[IBIS VER]   4.1
[File Name]   f28p55xpbk.ibs
[File Rev]   2.0
[Date]   August 28, 2024
[Source]   File originated at Texas Instruments
[Copyright]   (c) 2012, Texas Instruments Inc.
[Component]   f28p55xpbk
[Manufacturer]  Texas Instruments
[Package]
| Variable   Typ   Min   Max
R_pkg  3.39E-01  1.39E-01  3.88E-01
L_pkg  6.91E-09  4.87E-09  8.02E-09
C_pkg  9.61E-15  7.42E-15  1.07E-14
[Pin]   signal_name   model_name   R_pin   L_pin   C_pin
   1   GPIO29   BCF3385DSHYPBFZ_LC  3.76E-01  7.81E-09  1.01E-14
   2   A16,B16,C16,GPIO28   BCF3385DSHYPBFZ_LC  3.69E-01  7.66E-09  9.95E-15
   3   XRSn   BQ0491FS_USF  3.59E-01  7.49E-09  9.73E-15
   4   GPIO46   BCF3385DSHYPBFZ_LC  3.51E-01  7.33E-09  9.53E-15
   5   VDDIO   NC  3.49E-01  7.23E-09  9.37E-15
   6   VDD   NC  1.87E-01  5.49E-09  8.01E-15
   7   VSS   NC  1.86E-01  5.40E-09  7.86E-15
   8   GPIO47   BCF3385DSHYPBFZ_LC_USF  3.37E-01  6.88E-09  8.87E-15
   9   GPIO66   BCF3385DSHYPBFZ_LC_USF  3.33E-01  6.76E-09  1.03E-14
   10   GPIO67   BCF3385DSHYPBFZ_LC_USF  3.30E-01  6.66E-09  1.01E-14
   11   GPIO48   BCF3385DSHYPBFZ_LC_USF  3.28E-01  6.57E-09  9.90E-15
   12   GPIO49   BCF3385DSHYPBFZ_LC_USF  3.27E-01  6.48E-09  9.72E-15
   13   GPIO50   BCF3385DSHYPBFZ_LC_USF  3.27E-01  6.41E-09  9.55E-15
   14   GPIO51   BCF3385DSHYPBFZ_LC_USF  3.29E-01  6.35E-09  9.38E-15
   15   GPIO52   BCF3385DSHYPBFZ_LC_USF  3.31E-01  6.29E-09  9.22E-15
   16   GPIO53   BCF3385DSHYPBFZ_LC_USF  3.34E-01  6.25E-09  9.07E-15
   17   GPIO54   BCF3385DSHYPBFZ_LC_USF  3.36E-01  6.27E-09  9.09E-15
   18   A6,D14,E14,GPIO228   BCF3385DSHYPBFZ_LC_USF  3.36E-01  6.35E-09  9.26E-15
   19   B2,C6,E12,GPIO226   BCF3385DSHYPBFZ_LC_USF  3.37E-01  6.44E-09  9.45E-15
   20   A3,B3,C5,GPIO242,PGA2_INP   BCF3385DSHYPBFZ_LC_USF  3.58E-01  6.72E-09  9.78E-15
   21   A2,B6,C9,GPIO224,PGA1_INP   BCF3385DSHYPBFZ_LC  3.37E-01  6.58E-09  9.79E-15
   22   A15,B9,C7,PGA1_INM   ICF33SHYPB_LC  3.31E-01  6.59E-09  9.92E-15
   23   C25,D5,E5   ICF33SHYPB_LC  3.29E-01  6.65E-09  1.01E-14
   24   A26,D6,E6   ICF33SHYPB_LC  3.32E-01  6.76E-09  1.03E-14
   25   B26,D7,E7   ICF33SHYPB_LC  3.36E-01  6.87E-09  8.86E-15
   26   A14,B14,C4,PGA1_OUT   ICF33SHYPB_LC  3.40E-01  6.99E-09  9.03E-15
   27   A11,B10,C0,PGA2_OUT   ICF33SHYPB_LC  3.46E-01  7.13E-09  9.22E-15
   28   A5,B12,C2,PGA2_INM   ICF33SHYPB_LC  3.62E-01  7.36E-09  9.47E-15
   29   A1,B7,D11,DACB_OUT   ICF33SHYPB_LC  3.58E-01  7.39E-09  9.58E-15
   30   A0,B15,C15,DACA_OUT   ICF33SHYPB_LC  3.67E-01  7.56E-09  9.79E-15
   31   D20,E20,VREFHI   ICF33SHYPB_LC  3.73E-01  7.70E-09  9.97E-15
   32   D20,E20,VREFHI   ICF33SHYPB_LC  2.06E-01  6.06E-09  8.85E-15
   33   A13,B13,C13,D13,E13,VREFLO   ICF33SHYPB_LC  3.84E-01  8.02E-09  1.04E-14
   34   A13,B13,C13,D13,E13,VREFLO   ICF33SHYPB_LC  2.04E-01  6.08E-09  8.91E-15
   35   A12,C1,E11,PGA3_INP   ICF33SHYPB_LC  3.74E-01  7.75E-09  1.01E-14
   36   B11,D16,E16,PGA3_INM   ICF33SHYPB_LC  3.70E-01  7.63E-09  9.88E-15
   37   A7,B30,C3,D12,E30   ICF33SHYPB_LC  3.66E-01  7.52E-09  9.71E-15
   38   B5,D15,E15,PGA3_OUT   ICF33SHYPB_LC  3.69E-01  7.47E-09  9.59E-15
   39   A8,B0,C11   ICF33SHYPB_LC  3.59E-01  7.29E-09  9.37E-15
   40   VSSA   NC  1.40E-01  4.96E-09  7.57E-15
   41   VDDA   NC  1.39E-01  4.87E-09  7.42E-15
   42   A4,B8,C14   ICF33SHYPB_LC  3.65E-01  7.13E-09  1.06E-14
   43   C26,D8,E8,GPIO211   BCF3385DSHYPBFZ_LC  3.75E-01  7.15E-09  1.05E-14
   44   A27,D9,E9,GPIO212   BCF3385DSHYPBFZ_LC  3.71E-01  7.03E-09  1.03E-14
   45   B27,D10,E10,GPIO213   BCF3385DSHYPBFZ_LC  3.67E-01  6.91E-09  1.01E-14
   46   C27,D18,E18,GPIO214   BCF3385DSHYPBFZ_LC  3.65E-01  6.81E-09  9.87E-15
   47   A28,D19,E19,GPIO215   BCF3385DSHYPBFZ_LC  3.63E-01  6.72E-09  9.67E-15
   48   A9,GPIO227   BCF3385DSHYPBFZ_LC  3.62E-01  6.63E-09  9.49E-15
   49   B4,C8,GPIO236   BCF3385DSHYPBFZ_LC  3.60E-01  6.60E-09  9.47E-15
   50   A10,B1,C10,GPIO230   BCF3385DSHYPBFZ_LC  3.56E-01  6.65E-09  9.62E-15
   51   GPIO55   BCF3385DSHYPBFZ_LC  3.54E-01  6.70E-09  9.78E-15
   52   GPIO60   BCF3385DSHYPBFZ_LC  3.51E-01  6.75E-09  9.94E-15
   53   VSS   NC  1.90E-01  5.17E-09  8.90E-15
   54   VDD   NC  1.89E-01  5.24E-09  9.07E-15
   55   VDDIO   NC  3.51E-01  6.98E-09  1.05E-14
   56   GPIO64   BCF3385DSHYPBFZ_LC  3.46E-01  7.00E-09  8.99E-15
   57   GPIO65   BCF3385DSHYPBFZ_LC  3.47E-01  7.09E-09  9.14E-15
   58   GPIO62   BCF3385DSHYPBFZ_LC  3.49E-01  7.19E-09  9.30E-15
   59   GPIO63   BCF3385DSHYPBFZ_LC  3.52E-01  7.29E-09  9.46E-15
   60   A17,B17,C17,GPIO20   BCF3385DSHYPBFZ_LC  3.56E-01  7.42E-09  9.64E-15
   61   A18,B18,C18,GPIO21   BCF3385DSHYPBFZ_LC  3.61E-01  7.55E-09  9.82E-15
   62   A19,B19,C19,GPIO13   BCF3385DSHYPBFZ_LC  3.68E-01  7.69E-09  1.00E-14
   63   A20,B20,C20,GPIO12   BCF3385DSHYPBFZ_LC  3.76E-01  7.85E-09  1.02E-14
   64   A24,D0,E0,GPIO11   BCF3385DSHYPBFZ_LC  3.81E-01  7.98E-09  1.04E-14
   65   B24,D1,E1,GPIO33   BCF3385DSHYPBFZ_LC  3.80E-01  7.85E-09  1.02E-14
   66   C24,D2,E2,GPIO16   BCF3385DSHYPBFZ_LC  3.69E-01  7.66E-09  9.94E-15
   67   A25,D3,E3,GPIO17   BCF3385DSHYPBFZ_LC  3.60E-01  7.49E-09  9.73E-15
   68   B25,D4,E4,GPIO24   BCF3385DSHYPBFZ_LC  3.51E-01  7.33E-09  9.54E-15
   69   GPIO25   BCF3385DSHYPBFZ_LC  3.48E-01  7.22E-09  9.37E-15
   70   GPIO26   BCF3385DSHYPBFZ_LC  3.42E-01  7.08E-09  9.18E-15
   71   GPIO27   BCF3385DSHYPBFZ_LC  3.40E-01  6.98E-09  9.03E-15
   72   GPIO68   BCF3385DSHYPBFZ_LC  3.36E-01  6.87E-09  8.86E-15
   73   GPIO69   BCF3385DSHYPBFZ_LC  3.33E-01  6.76E-09  1.03E-14
   74   GPIO70   BCF3385DSHYPBFZ_LC  3.31E-01  6.67E-09  1.01E-14
   75   TCK   BCF3355DSHYPBFZ_TMS_USF  3.30E-01  6.59E-09  9.92E-15
   76   GPIO37/TDO   BCPF335585DSHYPBFZ  3.30E-01  6.52E-09  9.74E-15
   77   TMS   BCF3355DSHYPBFZ_TMS  3.32E-01  6.45E-09  9.58E-15
   78   GPIO35/TDI   BCF3385DSHYPBFZ_LC  3.34E-01  6.40E-09  9.42E-15
   79   GPIO32   BQ33100HYPBFZ_PMB_5FS_LC  3.36E-01  6.35E-09  9.27E-15
   80   GPIO56   BCF3385DSHYPBFZ_LC  3.39E-01  6.30E-09  9.11E-15
   81   GPIO57   BCF3385DSHYPBFZ_LC  3.41E-01  6.32E-09  9.12E-15
   82   GPIO58   BCF3385DSHYPBFZ_LC  3.41E-01  6.40E-09  9.30E-15
   83   GPIO71   BCF3385DSHYPBFZ_LC  3.42E-01  6.49E-09  9.49E-15
   84   GPIO72   BCF3385DSHYPBFZ_LC  3.45E-01  6.59E-09  9.68E-15
   85   GPIO73   BCF3385DSHYPBFZ_LC  3.48E-01  6.69E-09  9.87E-15
   86   GPIO74   BCF3385DSHYPBFZ_LC  3.52E-01  6.81E-09  1.01E-14
   87   GPIO18,X2   BCF3385DSHYPBFZ_LC  3.66E-01  7.03E-09  1.04E-14
   88   GPIO19,X1   BCPF335585DSHYPBFZ  3.51E-01  6.95E-09  1.04E-14
   89   VDDIO   NC  3.59E-01  7.11E-09  9.04E-15
   90   VDD   NC  1.89E-01  5.43E-09  7.88E-15
   91   GPIO43   BCF3385DSHYPBFZ_LC  3.54E-01  7.21E-09  9.28E-15
   92   VSS   NC  1.41E-01  5.09E-09  7.80E-15
   93   VREGENZ   IQ0440FS_VREGENZ_USF  3.58E-01  7.40E-09  9.58E-15
   94   GPIO42   BCF3385DSHYPBFZ_LC  3.67E-01  7.56E-09  9.79E-15
   95   GPIO8   BCF3385DSHYPBFZ_LC  3.77E-01  7.74E-09  1.00E-14
   96   GPIO4   BCF3385DSHYPBFZ_LC  3.80E-01  7.85E-09  1.02E-14
   97   GPIO3  BQ33100HYPBFZ_PMB_5FS_LC  3.85E-01  8.02E-09  1.04E-14
   98   GPIO2  BQ33100HYPBFZ_PMB_5FS_LC  3.87E-01  7.97E-09  1.03E-14
   99   GPIO1   BCF3385DSHYPBFZ_LC  3.85E-01  7.87E-09  1.01E-14
   100   GPIO0   BCF3385DSHYPBFZ_LC  3.78E-01  7.71E-09  9.94E-15
   101   GPIO40   BCF3385DSHYPBFZ_LC  3.70E-01  7.56E-09  9.74E-15
   102   GPIO23,USB0DM   NC  3.69E-01  7.47E-09  9.59E-15
   103   GPIO41,USB0DP   NC  3.65E-01  7.35E-09  9.42E-15
   104   GPIO22   BCF3385DSHYPBFZ_LC  3.64E-01  7.27E-09  9.27E-15
   105   GPIO7   BCF3385DSHYPBFZ_LC  3.60E-01  7.15E-09  9.10E-15
   106   GPIO44   BCF3385DSHYPBFZ_LC  3.72E-01  7.19E-09  1.06E-14
   107   VSS   NC  2.00E-01  5.35E-09  9.15E-15
   108   VDD   NC  2.04E-01  5.31E-09  9.00E-15
   109   VDDIO   NC  3.88E-01  7.12E-09  1.02E-14
   110   GPIO45   BCF3385DSHYPBFZ_LC  3.70E-01  6.87E-09  9.91E-15
   111   GPIO75   BCF3385DSHYPBFZ_LC  3.68E-01  6.76E-09  9.71E-15
   112   GPIO76   BCF3385DSHYPBFZ_LC  3.66E-01  6.66E-09  9.51E-15
   113   GPIO77   BCF3385DSHYPBFZ_LC  3.62E-01  6.63E-09  9.49E-15
   114   GPIO78   BCF3385DSHYPBFZ_LC  3.58E-01  6.66E-09  9.63E-15
   115   GPIO79   BCF3385DSHYPBFZ_LC  3.54E-01  6.70E-09  9.78E-15
   116   GPIO80   BCF3385DSHYPBFZ_LC  3.51E-01  6.75E-09  9.94E-15
   117   GPIO81   BCF3385DSHYPBFZ_LC  3.49E-01  6.81E-09  1.01E-14
   118   GPIO5   BCF3385DSHYPBFZ_LC  3.48E-01  6.87E-09  1.03E-14
   119   GPIO9  BQ33100HYPBFZ_PMB_5FS_LC  3.48E-01  6.95E-09  1.05E-14
   120   GPIO61   BCF3385DSHYPBFZ_LC_USF  3.45E-01  7.00E-09  8.98E-15
   121   GPIO59   BCF3385DSHYPBFZ_LC_USF  3.46E-01  7.08E-09  9.13E-15
   122   GPIO10   BCF3385DSHYPBFZ_LC_USF  3.48E-01  7.18E-09  9.29E-15
   123   GPIO34   BCF3385DSHYPBFZ_LC_USF  3.51E-01  7.29E-09  9.45E-15
   124   GPIO15   BCF3385DSHYPBFZ_LC_USF  3.55E-01  7.40E-09  9.63E-15
   125   GPIO14   BCF3385DSHYPBFZ_LC_USF  3.57E-01  7.51E-09  9.79E-15
   126   GPIO6   BCF3385DSHYPBFZ_LC_USF  3.64E-01  7.65E-09  9.98E-15
   127   GPIO30   BCF3385DSHYPBFZ_LC  3.71E-01  7.80E-09  1.02E-14
   128   GPIO31   BCF3385DSHYPBFZ_LC  3.85E-01  8.02E-09  1.04E-14
| End of package information
|   Component BQ0491FS_USF
[Component]   BQ0491FS_USF
[Manufacturer]   Texas Instruments
[Package]
|  variable   typ   min   max
R_pkg   0   0   0
L_pkg   0   0   0
C_pkg   0   0   0
[Pin]   signal_name   model_name   R_pin   L_pin   C_pin
VSS   VSS   GND
VDDS   VDDS   POWER
PAD   PAD   BQ0491FS_USF
[Model Selector] BQ0491FS_USF
WK_PU_ON_WITH_RX_3P3  Cell operated at 3.3(nom)
|WK_PU_ON_WITH_RX_3P3; WEAK_PULLUP_ON_WITH_RX
OPEN_DRAIN_MODE_3P3  Cell operated at 3.3(nom)
|   Component BCPF335585DSHYPBFZ
[Component]   BCPF335585DSHYPBFZ
[Manufacturer]   Texas Instruments
[Package]
|  variable   typ   min   max
R_pkg   0   0   0
L_pkg   0   0   0
C_pkg   0   0   0
[Pin]   signal_name   model_name   R_pin   L_pin   C_pin
VSS   VSS   GND
VDDS   VDDS   POWER
PAD   PAD   BCPF335585DSHYPBFZ
[Model Selector] BCPF335585DSHYPBFZ
BCPF_WK_PU_ON_3P3  Cell operated at 3.3(nom)
|BCPF_WK_PU_ON_3P3; WEAK_PULLUP_ON
BCPF_DRIVER_MODE_4MA_3P3  Cell operated at 3.3(nom)
|BCPF_DRIVER_MODE_4MA_3P3
BCPF_DRIVER_MODE_2MA_3P3  Cell operated at 3.3(nom)
|BCPF_DRIVER_MODE_2MA_3P3
BCPF_WK_PD_ON_3P3  Cell operated at 3.3(nom)
|   Component ICF33SHYPB_LC
[Component]   ICF33SHYPB_LC
[Manufacturer]   Texas Instruments
[Package]
|  variable   typ   min   max
R_pkg   0   0   0
L_pkg   0   0   0
C_pkg   0   0   0
[Pin]   signal_name   model_name   R_pin   L_pin   C_pin
VSS   VSS   GND
VDDS   VDDS   POWER
PAD   PAD   ICF33SHYPB_LC
[Model Selector] ICF33SHYPB_LC
ICF_RECEIVER_MODE_3P3  Cell operated at 3.3(nom)
|ICF_RECEIVER_MODE_3P3; RECEIVER_MODE
ICF_WK_PU_ON_3P3  Cell operated at 3.3(nom)
|ICF_WK_PU_ON_3P3; WEAK_PULLUP_ON
ICF_WK_PD_ON_3P3  Cell operated at 3.3(nom)
|   Component BCF3385DSHYPBFZ_LC_USF
[Component]   BCF3385DSHYPBFZ_LC_USF
[Manufacturer]   Texas Instruments
[Package]
|  variable   typ   min   max
R_pkg   0   0   0
L_pkg   0   0   0
C_pkg   0   0   0
[Pin]   signal_name   model_name   R_pin   L_pin   C_pin
VSS   VSS   GND
VDDS   VDDS   POWER
PAD   PAD   BCF3385DSHYPBFZ_LC_USF
[Model Selector] BCF3385DSHYPBFZ_LC_USF
BCF_WK_PU_ON_3P3  Cell operated at 3.3(nom)
|BCF_WK_PU_ON_3P3; WEAK_PULLUP_ON
BCF_WK_PD_ON_3P3  Cell operated at 3.3(nom)
|BCF_WK_PD_ON_3P3; WEAK_PULLDOWN_ON
BCF_DRIVER_MODE_3P3  Cell operated at 3.3(nom)
|BCF_DRIVER_MODE_3P3
BCF_RECEIVER_MODE_3P3  Cell operated at 3.3(nom)
|   Component BCF3355DSHYPBFZ_TMS_USF
[Component]   BCF3355DSHYPBFZ_TMS_USF
[Manufacturer]   Texas Instruments
[Package]
|  variable   typ   min   max
R_pkg   0   0   0
L_pkg   0   0   0
C_pkg   0   0   0
[Pin]   signal_name   model_name   R_pin   L_pin   C_pin
VSS   VSS   GND
VDDS   VDDS   POWER
PAD   PAD   BCF3355DSHYPBFZ_TMS_USF
[Model Selector] BCF3355DSHYPBFZ_TMS_USF
TMS_WK_PU_ON_3P3  Cell operated at 3.3(nom)
|TMS_WK_PU_ON_3P3; WEAK_PULLUP_ON
TMS_DRIVER_3P3  Cell operated at 3.3(nom)
|TMS_DRIVER_3P3
TMS_WK_PD_ON_3P3  Cell operated at 3.3(nom)
|   Component BCF3385DSHYPBFZ_LC
[Component]   BCF3385DSHYPBFZ_LC
[Manufacturer]   Texas Instruments
[Package]
|  variable   typ   min   max
R_pkg   0   0   0
L_pkg   0   0   0
C_pkg   0   0   0
[Pin]   signal_name   model_name   R_pin   L_pin   C_pin
VSS   VSS   GND
VDDS   VDDS   POWER
PAD   PAD   BCF3385DSHYPBFZ_LC
[Model Selector] BCF3385DSHYPBFZ_LC
BCF_WK_PU_ON_3P3  Cell operated at 3.3(nom)
|BCF_WK_PU_ON_3P3; WEAK_PULLUP_ON
BCF_WK_PD_ON_3P3  Cell operated at 3.3(nom)
|BCF_WK_PD_ON_3P3; WEAK_PULLDOWN_ON
BCF_DRIVER_MODE_3P3  Cell operated at 3.3(nom)
|BCF_DRIVER_MODE_3P3
BCF_RECEIVER_MODE_3P3  Cell operated at 3.3(nom)
|BCF_RECEIVER_MODE_3P3; RECEIVER_MODE
|   Component IQ0440FS_VREGENZ_USF
[Component]   IQ0440FS_VREGENZ_USF
[Manufacturer]   Texas Instruments
[Package]
|  variable   typ   min   max
R_pkg   0   0   0
L_pkg   0   0   0
C_pkg   0   0   0
[Pin]   signal_name   model_name   R_pin   L_pin   C_pin
VSS   VSS   GND
VDDS   VDDS   POWER
PAD   PAD   IQ0440FS_VREGENZ_USF
[Model Selector] IQ0440FS_VREGENZ_USF
VREGENZ_WK_PD_ON_3P3  Cell operated at 3.3(nom)
|VREGENZ_WK_PD_ON_3P3; WEAK_PULLDOWN_ON
VREGENZ_WK_PD_OFF_3P3  Cell operated at 3.3(nom)
|   Component BCF3355DSHYPBFZ_TMS
[Component]   BCF3355DSHYPBFZ_TMS
[Manufacturer]   Texas Instruments
[Package]
|  variable   typ   min   max
R_pkg   0   0   0
L_pkg   0   0   0
C_pkg   0   0   0
[Pin]   signal_name   model_name   R_pin   L_pin   C_pin
VSS   VSS   GND
VDDS   VDDS   POWER
PAD   PAD   BCF3355DSHYPBFZ_TMS
[Model Selector] BCF3355DSHYPBFZ_TMS
TMS_WK_PU_ON_3P3  Cell operated at 3.3(nom)
|TMS_WK_PU_ON_3P3; WEAK_PULLUP_ON
TMS_DRIVER_3P3  Cell operated at 3.3(nom)
|TMS_DRIVER_3P3
TMS_WK_PD_ON_3P3  Cell operated at 3.3(nom)
|TMS_WK_PD_ON_3P3; WEAK_PULLDOWN_ON
|   Component BQ33100HYPBFZ_PMB_5FS_LC
[Component]   BQ33100HYPBFZ_PMB_5FS_LC
[Manufacturer]  Texas Instruments
[Package]
| variable   typ   min   max
R_pkg   0.0   0.0   0.0
L_pkg   0.0H   0.0H   0.0H
C_pkg   0.0F   0.0F   0.0F
[Pin]  signal_name   model_name   R_pin   L_pin   C_pin
Pin1   PAD   BQ33100HYPBFZ_PMB_5FS_LC   0   0   0
Pin2   VDDS   Power   0   0   0
Pin3   VSS   Gnd   0   0   0
[Model Selector]   BQ33100HYPBFZ_PMB_5FS_LC
BQ33_PMB_IO_M0_D0   I/O model with Mode = 0 and Drive = 0
BQ33_PMB_IO_M0_D1   I/O model with Mode = 0 and Drive = 1
BQ33_PMB_IO_M1_D0   I/O model with Mode = 1 and Drive = 0
BQ33_PMB_IO_M1_D1   I/O model with Mode = 1 and Drive = 1
| Models and submodels in the file (22): WK_PU_ON_WITH_RX_3P3 (Input), OPEN_DRAIN_MODE_3P3 (I/O_open_drain), BCPF_WK_PU_ON_3P3 (Input), BCPF_DRIVER_MODE_4MA_3P3 (I/O), BCPF_DRIVER_MODE_2MA_3P3 (I/O), BCPF_WK_PD_ON_3P3 (Input), ICF_RECEIVER_MODE_3P3 (Input), ICF_WK_PU_ON_3P3 (Input), ICF_WK_PD_ON_3P3 (Input), BCF_WK_PU_ON_3P3 (Input), BCF_WK_PD_ON_3P3 (Input), BCF_DRIVER_MODE_3P3 (I/O), BCF_RECEIVER_MODE_3P3 (Input), TMS_WK_PU_ON_3P3 (Input), TMS_DRIVER_3P3 (I/O), TMS_WK_PD_ON_3P3 (Input), VREGENZ_WK_PD_ON_3P3 (Input), VREGENZ_WK_PD_OFF_3P3 (Input), BQ33_PMB_IO_M0_D0 (I/O), BQ33_PMB_IO_M0_D1 (I/O), BQ33_PMB_IO_M1_D0 (I/O), BQ33_PMB_IO_M1_D1 (I/O)
